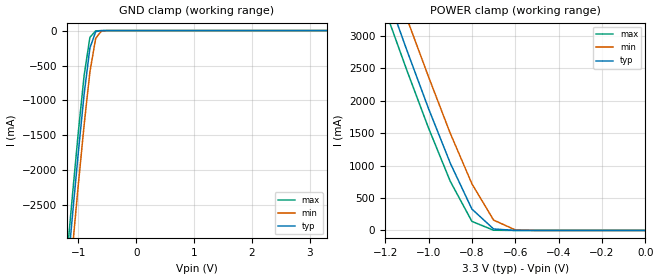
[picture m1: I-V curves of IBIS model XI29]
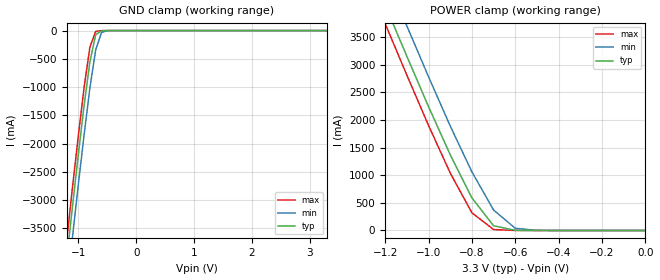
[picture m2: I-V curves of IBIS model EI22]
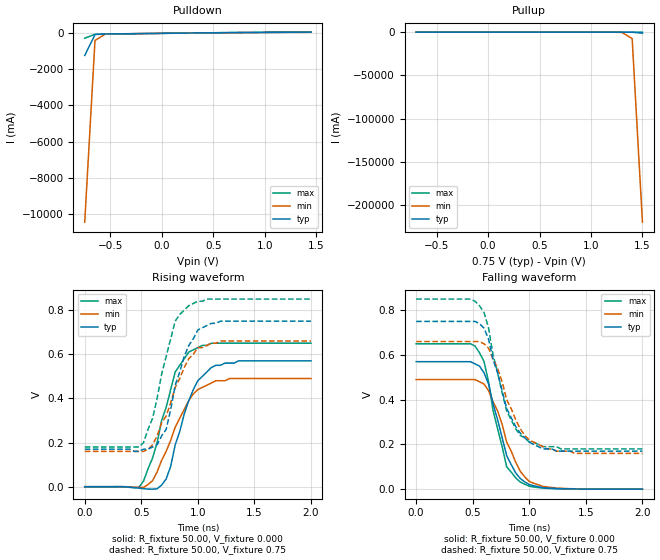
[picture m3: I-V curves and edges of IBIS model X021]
|   * 9dbl411a.ibs * IBIS 2.1 Model file
| Rev History
| Rev No.   Description
| 1.0   Initial release with Updated Parasitic Parameters
[IBIS Ver]   2.1
[Comment char]  |_char
[File name]   9dbl411a.ibs
[Date]   March 21, 2009
[File Rev]   1.0
[Source]   Originated at Integrated Circuit Systems, Inc.
[Disclaimer] (C) Copyright Integrated Circuit Systems, Inc. 2007
   All rights reserved
ICS hereby grants the user of this IBIS model a non-exclusive,
nontransferable license to use this IBIS model under the following terms.
Before using this IBIS model, the user should read this license.
If the user does not accept these terms,  the IBIS model should be
returned to ICS within 30 days.
   The user is granted this license only to use the IBIS model and
is not granted rights to sell, load, rent, lease or license the IBIS
model in whole or in part, or in modified form to anyone other than
user. User may modify the IBIS model to suit its specific
applications but rights to derivative works and such modifications
shall belong to ICS.
   This IBIS model is provided on an "AS IS" basis and ICS makes
absolutely no warranty with respect to the information contained
herein. ICS DISCLAIMS AND CUSTOMER WAIVES ALL WARRANTIES, EXPRESS
OR IMPLIED, INCLUDING WARRANTIES OF MERCHANTABILITY OR FITNESS FOR
A PARTICULAR PURPOSE. The entire risk as to quality and performance
is with the Customer. ACCORDINGLY, IN NO EVENT SHALL THE COMPANY BE
LIABLE FOR ANY DAMAGES, WHETHER IN CONTRACT OR TORT,INCLUDING ANY
LOST PROFITS OR OTHER INCIDENTAL, CONSEQUENTIAL, EXEMPLARY, OR
PUNITIVE DAMAGES ARISING OUT OF THE USE OR APPLICATION OF THE IBIS
model provided in this package. Further, ICS reserves the right to
make changes without notice to any product herein to improve
reliability, function, or design. ICS does not convey any license
under patent rights or any other intellectual property rights,
including those of third parties.
   ICS is not obligated to provide maintenance or support
for the licensed IBIS model.
|   COMPONENT: ICS9DBL411_MLF
[Component]   ICS9DBL411_MLF
[Manufacturer]  ICS
[Package]
| variable   typ   min   max
R_pkg   81.1m   62.2m   100.0m
L_pkg   6.7nH   4.9nH   8.5nH
C_pkg   0.53pF  0.21pF  0.85pF
[Pin]   signal_name   model_name   R_pin   L_pin   C_pin
1   VDDA   POWER
2   GNDA   GND
3   OE3#   XI29
4   DIF3C_LPR   X021
5   DIF3T_LPR   X021
6   VDD_IO   POWER
7   GND   GND
8   DIF2C_LPR   X021
9   DIF2T_LPR   X021
10   OE2#   XI29
11   DIF1C_LPR   X021
12   DIF1T_LPR   X021
13   OE1#   XI29
14   GND   GND
15   VDD_IO   POWER
16   DIF0C_LPR   X021
17   DIF0T_LPR   X021
18   OE0#   XI29
19   DIF_INC   EI22
20   DIF_INT   EI22
|** All model are simulated with typical corner process
[Diff Pin]   inv_pin   vdiff   tdelay_typ
5   4   NA   NA
9   8   NA   NA
12   11   NA   NA
17   16   NA   NA
20   19   NA   NA
|   COMPONENT: ICS9DBL411_TSSOP
[Component]   ICS9DBL411_TSSOP
[Manufacturer]  ICS
[Package]
| variable   typ   min   max
R_pkg   81.1m   62.2m   100.0m
L_pkg   6.7nH   4.9nH   8.5nH
C_pkg   0.53pF  0.21pF  0.85pF
[Pin]   signal_name   model_name   R_pin   L_pin   C_pin
1   OE0#   XI29
2   DIF_INC   EI22
3   DIF_INT   EI22
4   VDDA   POWER
5   GNDA   GND
6   OE3#   XI29
7   DIF3C_LPR   X021
8   DIF3T_LPR   X021
9   VDD_IO   POWER
10   GND   GND
11   DIF2C_LPR   X021
12   DIF2T_LPR   X021
13   OE2#   XI29
14   DIF1C_LPR   X021
15   DIF1T_LPR   X021
16   OE1#   XI29
17   GND   GND
18   VDD_IO   POWER
19   DIF0C_LPR   X021
20   DIF0T_LPR   X021
|** All model are simulated with typical corner process
[Diff Pin]   inv_pin   vdiff   tdelay_typ
3   2   NA   NA
8   7   NA   NA
12   11   NA   NA
15   14   NA   NA
20   19   NA   NA
| Models and submodels in the file (3): XI29 (Input), EI22 (Input), X021 (Output)
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|   Model XI29
[Model]   XI29
Model_type   Input
Vinl =   0.80V
Vinh =   2.00V
C_comp   3.40pF   2.85pF   3.95pF
[Temperature Range]   27.00   70.00   0.000
[Voltage Range]   3.30V   3.00V   3.70V
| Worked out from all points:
|   GND clamp passes 1 mA (typ) near -0.60 V on its own axis
|   POWER clamp passes 1 mA (typ) near -0.60 V on its own axis
[GND_clamp]
| voltage   I(typ)   I(min)   I(max)
-3.3V     -24.05A    -24.48A    -23.79A
-1.2V     -3.55A     -4.02A     -3.26A
-1.1V     -2.63A     -3.1A      -2.34A
-1V       -1.74A     -2.2A      -1.45A
-900mV    -910mA     -1.35A     -640mA
-800mV    -250mA     -590mA     -96.82mA
-700mV    -14.58mA   -110mA     -3.87mA
-600mV    -880uA     -5.82mA    -450uA
-500mV    -88.5uA    -350uA     -45.09uA
3.3V      130pA      470nA      90.8pA
[POWER_clamp]
| voltage   I(typ)   I(min)   I(max)
-3.3V     24.22A     24.67A     23.94A
-1.2V     3.71A      4.2A       3.4A
-1.1V     2.78A      3.27A      2.47A
-1V       1.88A      2.37A      1.58A
-900mV    1.04A      1.5A       760mA
-800mV    330mA      720mA      140mA
-700mV    23.1mA     160mA      3.86mA
-600mV    560uA      9.41mA     65.29uA
0V        130pA      310pA      130pA
|   Model EI22
[Model]   EI22
Model_type   Input
Polarity   Inverting
Vinl =   0.80V
Vinh =   2.00V
C_comp   3.40pF   2.85pF   3.95pF
[Temperature Range]   27.00   70.00   0.000
[Voltage Range]   3.30V   3.00V   3.70V
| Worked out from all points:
|   GND clamp passes 1 mA (typ) near -0.54 V on its own axis
|   POWER clamp passes 1 mA (typ) near -0.54 V on its own axis
[GND_clamp]
| voltage   I(typ)   I(min)   I(max)
-3.3V     -24.56A    -25.06A    -24.25A
-1.2V     -4.03A     -4.57A     -3.7A
-1.1V     -3.1A      -3.64A     -2.76A
-1V       -2.19A     -2.72A     -1.86A
-900mV    -1.32A     -1.84A     -1A
-800mV    -550mA     -1.01A     -290mA
-700mV    -72.98mA   -340mA     -14.72mA
-600mV    -2.31mA    -32.86mA   -440uA
-500mV    -87.34uA   -1.32mA    -27.68uA
3.3V      71.49pA    1.81uA     53.65pA
[POWER_clamp]
| voltage   I(typ)   I(min)   I(max)
-3.3V     24.62A     25.13A     24.3A
-1.2V     4.08A      4.63A      3.74A
-1.1V     3.15A      3.7A       2.81A
-1V       2.24A      2.78A      1.9A
-900mV    1.37A      1.89A      1.04A
-800mV    590mA      1.06A      320mA
-700mV    85.08mA    370mA      16.78mA
-600mV    2.46mA     39.49mA    260uA
-500mV    53.03uA    1.53mA     3.94uA
0V        71.49pA    320pA      74.53pA
|   Model X021
[Model]   X021
Model_type   Output
Polarity   Non-Inverting
Vmeas =   0.37V
Vref =   0.37V
C_comp   3.40pF   2.85pF   3.95pF
[Temperature Range]   27.00   70.00   0.000
[Voltage Range]   0.75V   0.66V   0.85V
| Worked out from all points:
|   slope of the pulldown table from 0 to 0.112 V, typ, clamps not added: 14.2 ohm
|   slope of the pullup table from 0 to 0.112 V, typ, clamps not added: 15.6 ohm
|   rising waveform, R_fixture 50.00, V_fixture 0.000: 20-80 % time 207ps typ, 259ps min, 200ps max; typ from 0 V to 0.57 V
|   rising waveform, R_fixture 50.00, V_fixture 0.75: 20-80 % time 184ps typ, 240ps min, 181ps max; typ from 0.17 V to 0.75 V
|   falling waveform, R_fixture 50.00, V_fixture 0.000: 20-80 % time 190ps typ, 223ps min, 164ps max; typ from 0.57 V to 0 V
|   falling waveform, R_fixture 50.00, V_fixture 0.75: 20-80 % time 218ps typ, 233ps min, 195ps max; typ from 0.75 V to 0.17 V
[Pulldown]
| voltage   I(typ)   I(min)   I(max)
-750mV    -1.23A     -10.47A    -270mA
-650mV    -68.88mA   -390mA     -49.59mA
-550mV    -37.91mA   -46.36mA   -39.6mA
1.45V     65.77mA    60mA       69.66mA
[Pullup]
| voltage   I(typ)   I(min)   I(max)
-700mV    32.83mA    30.62mA    33.4mA
1.3V      -76.98mA   -320mA     -79.23mA
1.4V      -110mA     -7.51A     -84.56mA
1.5V      -1.27A     -220A      -93.1mA
[Ramp]
| variable   typ   min   max
dV/dt_r   0.34/0.21n   0.29/0.26n   0.39/0.21n
dV/dt_f   0.35/0.21n   0.30/0.23n   0.40/0.19n
R_load = 50.00
[Rising Waveform]
R_fixture = 50.00
V_fixture = 0.000
V_fixture_min = 0.000
V_fixture_max = 0.000
| time   V(typ)   V(min)   V(max)
0s        0V         0V         0V
480ps     -6.44mV    -3.56mV    -1.9mV
600ps     -11.2mV    27.28mV    130mV
720ps     35.15mV    160mV      360mV
760ps     92.37mV    210mV      440mV
800ps     190mV      270mV      520mV
920ps     390mV      390mV      610mV
1ns       480mV      440mV      630mV
1.16ns    550mV      480mV      650mV
2ns       570mV      490mV      650mV
[Rising Waveform]
R_fixture = 50.00
V_fixture = 0.75
V_fixture_min = 0.66
V_fixture_max = 0.85
| time   V(typ)   V(min)   V(max)
0s        170mV      160mV      180mV
480ps     160mV      160mV      180mV
520ps     170mV      160mV      200mV
600ps     180mV      190mV      310mV
720ps     260mV      320mV      590mV
800ps     460mV      450mV      750mV
920ps     640mV      580mV      820mV
1ns       710mV      630mV      840mV
1.2ns     750mV      660mV      850mV
2ns       750mV      660mV      850mV
[Falling Waveform]
R_fixture = 50.00
V_fixture = 0.000
V_fixture_min = 0.000
V_fixture_max = 0.000
| time   V(typ)   V(min)   V(max)
0s        570mV      490mV      650mV
520ps     560mV      490mV      640mV
600ps     520mV      470mV      570mV
640ps     470mV      440mV      480mV
680ps     380mV      390mV      350mV
760ps     230mV      290mV      190mV
800ps     150mV      210mV      100mV
920ps     47.74mV    79.85mV    31.95mV
1.12ns    6.84mV     12.26mV    4.78mV
2ns       29.38uV    57.85uV    25.96uV
[Falling Waveform]
R_fixture = 50.00
V_fixture = 0.75
V_fixture_min = 0.66
V_fixture_max = 0.85
| time   V(typ)   V(min)   V(max)
0s        750mV      660mV      850mV
480ps     750mV      660mV      850mV
560ps     740mV      660mV      820mV
640ps     670mV      630mV      720mV
680ps     580mV      580mV      600mV
800ps     360mV      400mV      350mV
920ps     250mV      270mV      240mV
1ns       210mV      220mV      210mV
1.4ns     170mV      160mV      180mV
2ns       170mV      160mV      180mV
